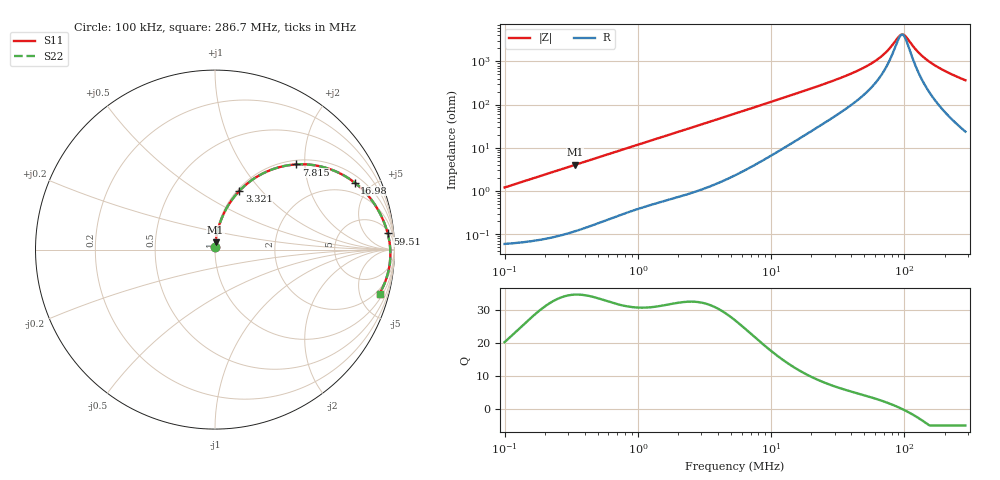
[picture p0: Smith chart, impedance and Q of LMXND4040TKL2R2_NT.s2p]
! LMXND4040TKL2R2_NT  S-PARAMETER MODEL  ( Standard Model )
! Model Generated by TAIYO YUDEN Corporation (https://www.yuden.co.jp/en/)
! Version 1.0
! TAIYO YUDEN Control No. 20250409
! Copyright(c) 2025 TAIYO YUDEN CO.,LTD. All Rights Reserved.
! Product Description (link to TY-COMPAS)
! https://ds.yuden.co.jp/TYCOMPAS/or/detail?pn=LMXND4040TKL2R2MNT&u=M
! Products Name : Inductors
! Characteristics :
!  Inductance : 2.2 [uH] , SRF(min) : 60 [MHz] , DC Resistance(max) : 0.0504 [Ohm]
!  Rated Current : Saturation  3000 [mA] , Temp Rise  2900 [mA] (40 [degC])
!  Case Size : 4.0 x 4.0 / 0.157 x 0.157 [mm/inch] , Thickness : 1.8 / 0.071 [mm/inch]
!  (Conditions: Temperature = 25 [degC] , DC Bias Current = 0 [A])
! External Node Assignments :
!  1  o---GGG---o  2
! GND o---------o GND
! Frequency Range : 0.1MHz  -  286.687601MHz  [ 402 STEP ]
# MHz S RI R 50
! Freq[MHz].  S11 Real  S11 Imag  S21 Real  S21 Imag  S12 Real  S12 Imag  S22 Real  S22 Imag
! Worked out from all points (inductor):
!   401 points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, 100 kHz to 286.7 MHz, reference 50 ohm
!   read as one part in series: L = 1.92 uH near 104.1 kHz
!   highest Q = 34.5 at 336.7 kHz (marker M1), where L = 1.91 uH
!   self-resonance near 95.81 MHz
!   S11 on the Smith chart (normalised r, x): 100 kHz: 1.00, +0.02; 3.321 MHz: 1.02, +0.77; 7.815 MHz: 1.09, +1.81; 16.98 MHz: 1.35, +3.96; 59.51 MHz: 7, +19; 286.7 MHz: 1.47, -7.29
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0.1  0.000744 0.0121  0.9993 -0.0121  0.9993 -0.0121  0.000744 0.0121
0.336709  0.00279 0.0402  0.9972 -0.0402  0.9972 -0.0402  0.00279 0.0402
0.379416  0.00337 0.0453  0.9966 -0.0453  0.9966 -0.0453  0.00337 0.0453
1.439567  0.0325 0.1619  0.9675 -0.1619  0.9675 -0.1619  0.0325 0.1619
3.320932  0.1363 0.3277  0.8637 -0.3277  0.8637 -0.3277  0.1363 0.3277
5.354322  0.284 0.4326  0.716 -0.4326  0.716 -0.4326  0.284 0.4326
7.815043  0.4518 0.4746  0.5482 -0.4746  0.5482 -0.4746  0.4518 0.4746
11.18188  0.6199 0.4551  0.3801 -0.4551  0.3801 -0.4551  0.6199 0.4551
16.98356  0.7782 0.3731  0.2218 -0.3731  0.2218 -0.3731  0.7782 0.3731
20.31517  0.8276 0.329  0.1724 -0.329  0.1724 -0.329  0.8276 0.329
39.1793  0.9326 0.1738  0.0674 -0.1738  0.0674 -0.1738  0.9326 0.1738
59.50735  0.9623 0.09  0.0377 -0.09  0.0377 -0.09  0.9623 0.09
68.40302  0.9684 0.0636  0.0316 -0.0636  0.0316 -0.0636  0.9684 0.0636
77.07906  0.9724 0.0411  0.0276 -0.0411  0.0276 -0.0411  0.9724 0.0411
90.38256  0.9759 0.0111  0.0241 -0.0111  0.0241 -0.0111  0.9759 0.0111
94.05279  0.9764 0.00354  0.0236 -0.00354  0.0236 -0.00354  0.9764 0.00354
97.87206  0.9768 -0.00405  0.0232 0.00405  0.0232 0.00405  0.9768 -0.00405
103.8937  0.9772 -0.0155  0.0228 0.0155  0.0228 0.0155  0.9772 -0.0155
129.3207  0.9757 -0.0589  0.0243 0.0589  0.0243 0.0589  0.9757 -0.0589
154.6891  0.9709 -0.0964  0.0291 0.0964  0.0291 0.0964  0.9709 -0.0964
204.3944  0.955 -0.1597  0.045 0.1597  0.045 0.1597  0.955 -0.1597
286.6876  0.9166 -0.2459  0.0834 0.2459  0.0834 0.2459  0.9166 -0.2459
